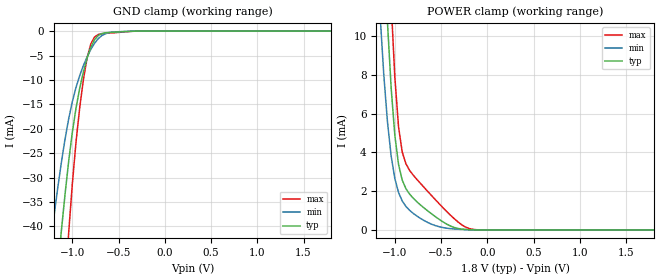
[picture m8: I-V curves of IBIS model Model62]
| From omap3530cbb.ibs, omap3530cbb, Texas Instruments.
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| Model based on original model for CSI2PHY3LANE_7LM
|   Sub model LPRX_DX2
[model]   Model62
|[Input Load]
|[Output Drive]
|Voltage   1.8V
|Mode   INPUT
Model_type   Input
Vinl =   0.55V
Vinh =   0.88V
C_comp   2.04pF 1.98pF 2.15pF
[Temperature Range]   27.00   125   -40
[Voltage Range]   1.8V   1.69V   1.92V
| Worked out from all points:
|   GND clamp passes 1 mA (typ) near -0.72 V on its own axis
|   POWER clamp passes 1 mA (typ) near -0.65 V on its own axis
[GND clamp]
-1.8V     -195.5mA   -140.4mA   -280.6mA
-1.24V    -66.24mA   -44.16mA   -102.2mA
-1.2V     -57.62mA   -38.15mA   -89.48mA
-1.12V    -41.2mA    -27.11mA   -64.56mA
-1.04V    -26.74mA   -18.03mA   -41.45mA
-960mV    -15.76mA   -11.52mA   -22.71mA
-880mV    -8.337mA   -7.047mA   -9.913mA
-840mV    -5.522mA   -5.272mA   -5.473mA
-800mV    -3.304mA   -3.75mA    -2.625mA
-720mV    -914.6uA   -1.561mA   -689.6uA
-400mV    -74.01uA   -55.49uA   -104.4uA
1.8V      821.4nA    1.764uA    1.336uA
[POWER_clamp]
-1.8V     115.8mA    92.28mA    137.7mA
-1.16V    19.65mA    11.15mA    28.05mA
-1.08V    10.76mA    5.599mA    16.62mA
-1.04V    7.349mA    3.824mA    11.77mA
-1V       4.888mA    2.656mA    7.888mA
-960mV    3.383mA    1.935mA    5.33mA
-920mV    2.571mA    1.496mA    4.018mA
-880mV    2.13mA     1.213mA    3.411mA
-720mV    1.278mA    588.4uA    2.387mA
-400mV    207.6uA    68.5uA     771uA
-160mV    6.77uA     5.748uA    33.75uA
1.8V      -511.5pA   -182.3nA   -301.2pA
